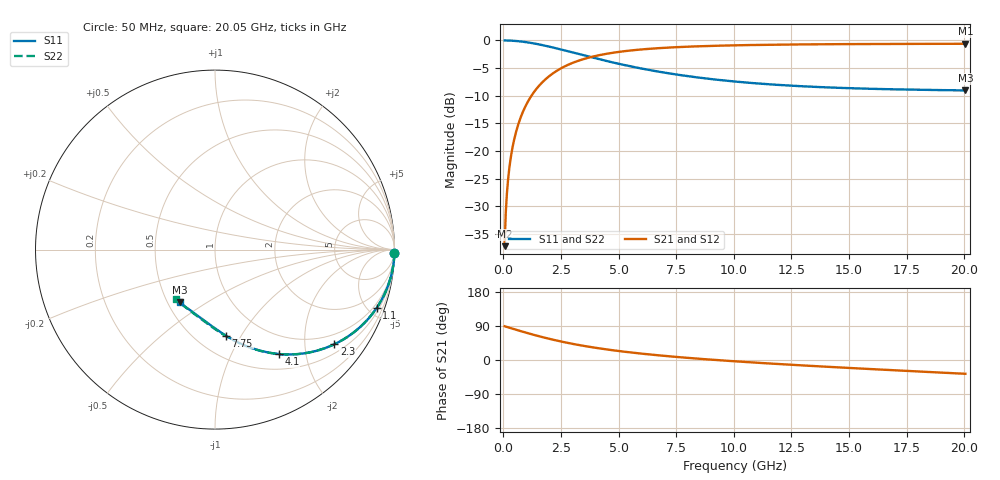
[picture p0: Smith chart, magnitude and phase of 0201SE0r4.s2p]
! AVX Thin Film Operation		Date: August 2001
! Description: Accu-P® Series, Thin Film, SMD, RF Capacitor
! Part Number: 02013J0R4ABW
! 50 MHz  -  20.05 GHz
! Serial Measurements
# mhz S db R 50
!	S11		S21		S12		S22
!	dB	Phase	dB	Phase	dB	Phase	dB	Phase
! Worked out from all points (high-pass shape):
!   401 points, 50 MHz to 20.05 GHz, reference 50 ohm
!   highest |S21| = -0.61 dB at 20.05 GHz (marker M1); lowest = -37.2 dB at 50 MHz (marker M2)
!   |S21| within 3 dB of the highest: 3.301 GHz to end of sweep
!   lowest |S11| = -9.0 dB at 20.05 GHz (marker M3), VSWR 2.09, Z = 28.8 - j19.3 ohm
!   |S11| at or under -10 dB: nowhere
!   |S22| runs from -9.1 to 0.0 dB; largest |S21 - S12| = 0
!   S11 on the Smith chart (normalised r, x): 50 MHz: open; 1.1 GHz: 0.72, -5.60; 2.3 GHz: 0.72, -2.70; 4.1 GHz: 0.71, -1.54; 7.75 GHz: 0.69, -0.86; 20.05 GHz: 0.58, -0.39
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50  -0.00 -0.9  -37.23 89.1  -37.23 89.1  -0.00 -0.9
100  -0.00 -1.9  -31.20 88.1  -31.20 88.1  -0.00 -1.9
200  -0.01 -3.7  -25.19 86.3  -25.19 86.3  -0.01 -3.7
250  -0.02 -4.6  -23.26 85.4  -23.26 85.4  -0.02 -4.7
300  -0.03 -5.6  -21.69 84.4  -21.69 84.4  -0.03 -5.6
400  -0.05 -7.4  -19.21 82.6  -19.21 82.6  -0.05 -7.4
550  -0.10 -10.2  -16.50 79.8  -16.50 79.8  -0.10 -10.2
700  -0.16 -12.9  -14.47 77.1  -14.47 77.1  -0.16 -12.9
900  -0.26 -16.4  -12.39 73.5  -12.39 73.5  -0.26 -16.4
1100  -0.38 -19.9  -10.78 70.1  -10.78 70.1  -0.38 -19.9
1650  -0.81 -28.9  -7.73 61.0  -7.73 61.0  -0.81 -29.0
2300  -1.43 -38.5  -5.53 51.5  -5.53 51.5  -1.43 -38.5
2800  -1.96 -44.9  -4.42 45.0  -4.42 45.0  -1.96 -45.0
3400  -2.60 -51.8  -3.47 38.2  -3.47 38.2  -2.60 -51.8
4100  -3.34 -58.6  -2.71 31.2  -2.71 31.2  -3.34 -58.7
5350  -4.54 -68.7  -1.89 21.1  -1.89 21.1  -4.54 -68.8
6750  -5.66 -77.5  -1.39 12.2  -1.39 12.2  -5.66 -77.8
7750  -6.31 -82.7  -1.17 6.9  -1.17 6.9  -6.32 -83.2
10050  -7.44 -92.7  -0.88 -3.5  -0.88 -3.5  -7.45 -93.7
13400  -8.38 -104.5  -0.70 -15.7  -0.70 -15.7  -8.40 -106.4
16750  -8.83 -114.6  -0.63 -26.5  -0.63 -26.5  -8.85 -117.6
20050  -9.04 -123.8  -0.60 -36.4  -0.60 -36.4  -9.07 -128.1
